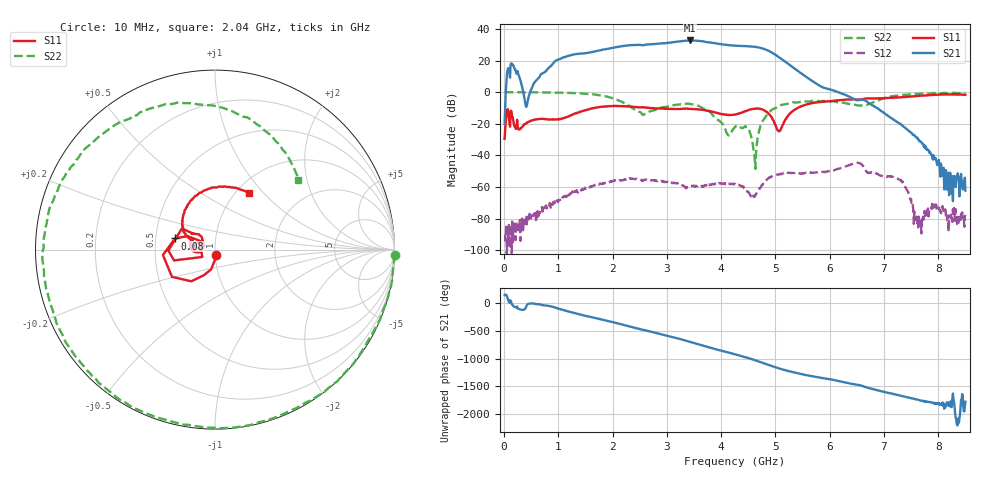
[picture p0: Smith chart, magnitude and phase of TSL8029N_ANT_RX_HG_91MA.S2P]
!Agilent Technologies,E5071C,MY46523237,B.13.01
!Date: Wed Aug 16 14:04:14 2023
!Data & Calibration Information:
!Freq	S11:SOLT2(ON)	S21:SOLT2(ON)	S12:SOLT2(ON)	S22:SOLT2(ON)
!PortZ  Port1:50+j0  Port2:50+j0
!Above PortZ is port z conversion or system Z0 setting when saving the data.
!When reading, reference impedance value at option line is always used.
# Hz S dB R 50
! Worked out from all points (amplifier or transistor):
!   850 points, 10 MHz to 8.5 GHz, reference 50 ohm
!   highest |S21| = 32.7 dB at 3.42 GHz (marker M1)
!   |S21| within 3 dB of that: 2.566 GHz to 4.153 GHz (1.587 GHz wide, 47.3 % of centre)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
!   unconditionally stable (mu >= 1): 18.53 MHz to 43.68 MHz; 67.98 MHz to 245.4 MHz; 253.9 MHz to end of sweep
!   at 1.42 GHz: K = 6.14, MAG = 32.3 dB, |S12| = -62.0 dB
!   at 4.26 GHz: K = 12.91, MAG = 29.6 dB, |S12| = -58.0 dB
!   at 8.5 GHz: K = 179866.09, MAG = -47.9 dB, |S12| = -77.6 dB
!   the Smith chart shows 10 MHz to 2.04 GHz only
!   S11 on the Smith chart (normalised r, x): 10 MHz: 1.01, -0.07; 80 MHz: 0.63, +0.08; 2.04 GHz: 1.15, +0.83
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1e7  -29.49 -76.3  -20.03 145.3  -90.28 -107.6  0.05 -1.7
8e7  -12.73 164.4  15.16 42.7  -87.89 35.1  -0.00 -15.5
1.05e9  -16.94 155.4  21.19 -112.3  -67.36 139.2  -0.32 -171.3
1.43e9  -12.12 136.6  24.46 146.4  -62.05 68.1  -0.87 138.1
1.76e9  -9.41 97.4  26.40 73.8  -57.87 6.8  -1.94 89.8
2.04e9  -8.76 59.0  28.29 7.5  -55.70 -41.3  -4.36 40.0
2.23e9  -8.89 32.4  29.27 -39.9  -55.30 -73.6  -7.19 -4.6
2.44e9  -9.41 3.5  29.89 -93.3  -54.86 -115.4  -11.60 -74.2
2.84e9  -10.26 -50.2  30.66 172.0  -56.09 -176.2  -10.28 167.1
3.17e9  -10.60 -95.7  31.81 91.2  -57.55 129.5  -8.00 111.1
3.42e9  -10.54 -134.6  32.68 22.2  -59.79 105.9  -7.37 67.7
3.57e9  -10.85 -160.1  32.49 -21.6  -59.14 86.7  -8.44 39.9
3.79e9  -12.03 156.1  31.37 -82.5  -58.81 59.5  -12.41 7.1
4.03e9  -13.86 98.1  30.13 -145.5  -57.72 12.1  -20.35 -3.4
4.26e9  -14.12 24.4  29.39 155.7  -58.02 -31.9  -21.68 35.8
4.5e9  -11.34 -53.8  29.00 88.0  -63.08 -126.9  -22.95 16.6
4.72e9  -10.53 -123.4  28.06 17.1  -60.30 63.1  -21.79 126.5
4.96e9  -17.69 150.2  24.48 -65.1  -52.70 -30.4  -10.65 78.5
5.2e9  -16.40 -39.1  18.82 -135.9  -50.91 -92.4  -7.56 31.3
5.67e9  -6.96 -129.1  7.28 119.7  -50.77 -177.8  -5.64 -39.8
7.09e9  -3.61 90.1  -15.33 177.1  -53.17 -114.7  -3.04 -16.6
8.5e9  -1.71 -102.9  -62.21 19.5  -77.63 -15.6  -0.52 -168.9
